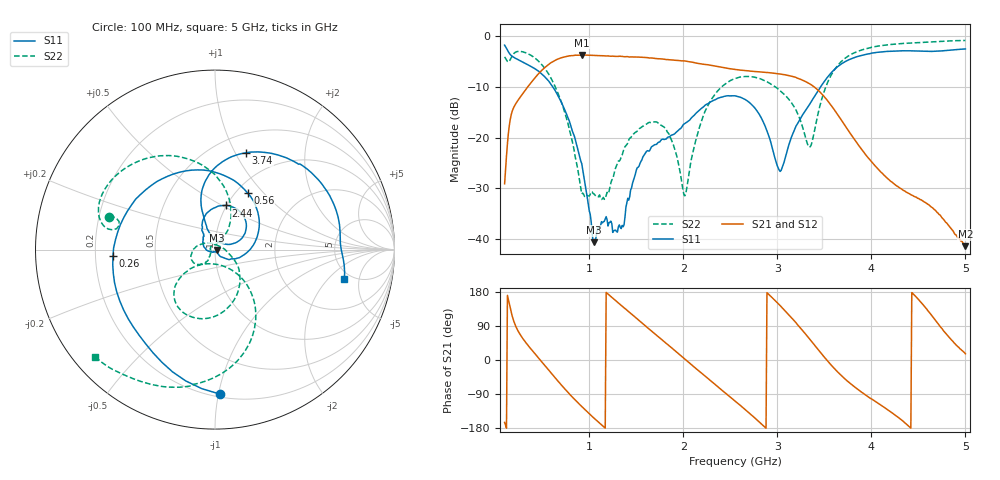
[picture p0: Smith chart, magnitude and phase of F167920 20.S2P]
!  2-Port S-parameters saved by WinCal
! VAR MeasName=S-Parameters (CALIBRATED_DATA) read from VNA (N5242A)
! VAR MeasDate=2016-11-22 9:56:09
! VAR NAME=F167920 20
! VAR FILENAME=F167920 20.S2P
! VAR DATE=2016-11-22 9:56:09
! VAR PHYS_PORTS=1,2
# Hz S DB R 50
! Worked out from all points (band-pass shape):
!   491 points, 100 MHz to 5 GHz, reference 50 ohm
!   highest |S21| = -3.80 dB at 920 MHz (marker M1); lowest = -41.3 dB at 5 GHz (marker M2)
!   |S21| within 3 dB of the highest: 496.7 MHz to 2.622 GHz (2.126 GHz wide, 136 % of centre)
!   lowest |S11| = -40.5 dB at 1.05 GHz (marker M3), VSWR 1.02, Z = 50.9 - j0.21 ohm
!   |S11| at or under -10 dB: 611.1 MHz to 3.463 GHz (2.852 GHz wide, 140 % of centre)
!   |S22| runs from -32.1 to -1.0 dB; largest |S21 - S12| = 0.0013
!   S11 on the Smith chart (normalised r, x): 100 MHz: 0.22, -1.01; 260 MHz: 0.27, -0.03; 560 MHz: 1.13, +0.82; 2.44 GHz: 1.00, +0.52; 3.74 GHz: 0.70, +1.11; 5 GHz: 4.32, -3.13
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1e8  -1.87 -87.9  -29.08 -164.7  -29.12 -164.7  -4.18 162.7
1.7e8  -3.90 -131.3  -15.55 126.0  -15.54 126.1  -4.34 169.1
2.6e8  -4.89 -176.3  -12.24 69.3  -12.24 69.3  -3.09 151.6
4.1e8  -6.37 118.5  -8.58 20.3  -8.58 20.3  -4.23 122.2
5.6e8  -8.78 60.0  -5.79 -24.0  -5.79 -24.1  -7.31 92.1
7.5e8  -15.02 -5.8  -4.12 -78.9  -4.12 -78.9  -15.71 59.9
9.2e8  -25.09 -48.5  -3.80 -122.7  -3.80 -122.6  -31.07 87.1
1.05e9  -40.55 -12.7  -3.89 -153.3  -3.89 -153.3  -31.06 147.8
1.35e9  -37.25 -121.8  -4.08 141.9  -4.08 141.9  -23.43 -123.7
1.44e9  -30.30 -156.4  -4.18 123.4  -4.18 123.4  -20.05 -129.9
1.74e9  -20.91 136.4  -4.55 60.3  -4.55 60.3  -17.21 -166.0
2.02e9  -17.22 120.8  -4.98 1.8  -4.99 1.8  -31.39 61.0
2.21e9  -14.05 105.8  -5.62 -37.7  -5.62 -37.8  -15.87 -36.6
2.44e9  -11.91 75.8  -6.31 -85.7  -6.33 -85.7  -9.58 -77.6
2.55e9  -11.82 59.9  -6.64 -108.2  -6.66 -108.2  -8.43 -93.4
2.81e9  -15.50 23.9  -7.12 -163.8  -7.13 -163.8  -8.42 -123.4
3.03e9  -26.66 63.3  -7.53 143.6  -7.53 143.6  -10.83 -138.6
3.37e9  -12.68 108.3  -9.78 47.2  -9.78 47.2  -20.85 -72.0
3.53e9  -8.24 97.8  -12.67 -1.3  -12.69 -1.3  -9.41 -51.5
3.74e9  -4.93 72.2  -18.22 -54.5  -18.26 -54.3  -4.20 -76.8
4.19e9  -3.08 29.5  -28.32 -134.1  -28.34 -134.0  -1.78 -110.5
5e9  -2.62 -12.8  -41.32 16.4  -41.22 17.5  -0.96 -138.3
